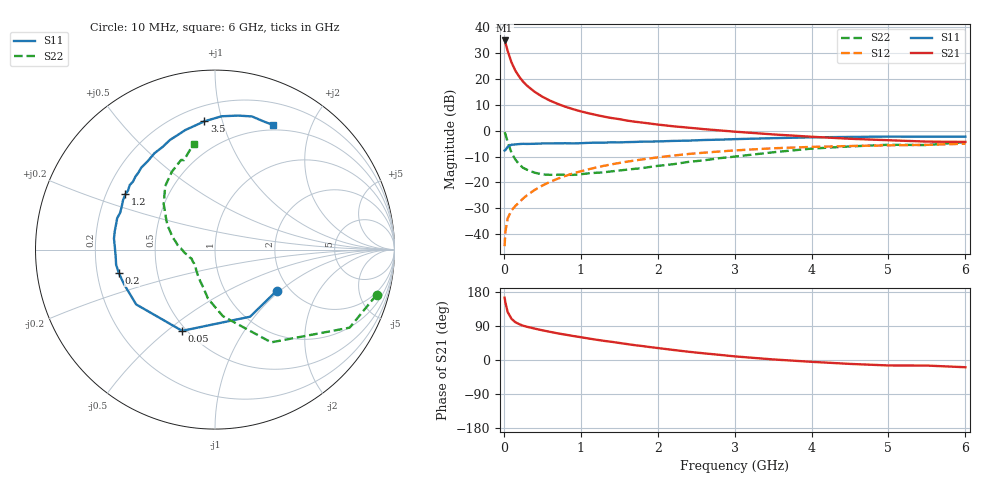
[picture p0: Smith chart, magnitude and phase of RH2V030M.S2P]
! SIEMENS Small Signal Semiconductors
! BFR106
! Si NPN RF Bipolar Junction Transistor in SOT23
! VCE = 2 V  IC = 30 mA
! Common Emitter S-Parameters:  August  1996
# GHz  S  MA  R  50
!  f  S11  S21  S12  S22
! GHz  MAG  ANG  MAG  ANG  MAG  ANG  MAG  ANG
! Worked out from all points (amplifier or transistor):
!   36 points, 10 MHz to 6 GHz, reference 50 ohm
!   highest |S21| = 35.0 dB at 10 MHz (marker M1)
!   |S21| within 3 dB of that: start of sweep to 40.17 MHz
!   unconditionally stable (mu >= 1): 287.5 MHz to 2.562 GHz; 5.108 GHz to end of sweep
!   at 250 MHz: K = 0.97, MSG = 22.6 dB, |S12| = -26.3 dB
!   at 1.4 GHz: K = 1.06, MAG = 7.4 dB, |S12| = -13.0 dB
!   at 6 GHz: K = 1.01, MAG = -0.3 dB, |S12| = -5.0 dB
!   S11 on the Smith chart (normalised r, x): 10 MHz: 1.71, -0.95; 50 MHz: 0.47, -0.56; 200 MHz: 0.29, -0.11; 1.2 GHz: 0.28, +0.26; 3.5 GHz: 0.30, +0.88; 6 GHz: 0.44, +1.48
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0.01  0.413 -33.9  56.01 164.5  0.0058 81.0  0.9349 -15.6
0.02  0.4219 -62.4  50.95 151.9  0.011 68.2  0.8671 -30.1
0.05  0.4882 -112.0  35.09 126.5  0.02 56.2  0.6041 -58.8
0.1  0.535 -145.2  20.98 108.5  0.0287 54.0  0.3729 -83.3
0.15  0.5421 -159.0  14.54 99.7  0.0349 57.1  0.2761 -98.1
0.2  0.5516 -166.2  11.12 94.6  0.0412 60.5  0.2223 -106.9
0.25  0.5573 -171.5  8.914 90.5  0.0485 62.5  0.191 -116.2
0.3  0.5547 -175.3  7.483 87.7  0.056 64.7  0.1755 -122.4
0.4  0.5584 178.4  5.679 82.9  0.0712 66.5  0.1539 -133.1
0.5  0.5664 173.7  4.561 78.4  0.0864 67.3  0.1425 -140.5
0.6  0.5679 169.3  3.827 74.3  0.1022 67.3  0.1397 -145.5
0.7  0.5691 165.3  3.309 70.3  0.1174 66.8  0.1404 -150.4
0.9  0.5669 158.7  2.613 63.4  0.149 65.1  0.1395 -158.7
1.1  0.5821 151.6  2.179 56.8  0.179 62.5  0.1493 -163.7
1.2  0.5865 148.3  2.017 53.6  0.1936 61.2  0.153 -166.9
1.6  0.6015 137.5  1.571 42.1  0.251 55.3  0.1759 -176.7
2.2  0.6342 122.1  1.219 26.6  0.3298 45.7  0.2242 168.5
2.8  0.6706 108.3  1.015 13.7  0.3955 35.9  0.2933 153.6
3.5  0.7172 94.7  0.848 1.5  0.4568 25.0  0.3822 138.4
4.5  0.7575 80.3  0.698 -10.3  0.5049 10.5  0.4964 118.9
5.5  0.7638 69.0  0.615 -14.7  0.5327 1.5  0.5275 109.1
6  0.7659 65.0  0.607 -19.1  0.5593 -5.3  0.6023 101.4
